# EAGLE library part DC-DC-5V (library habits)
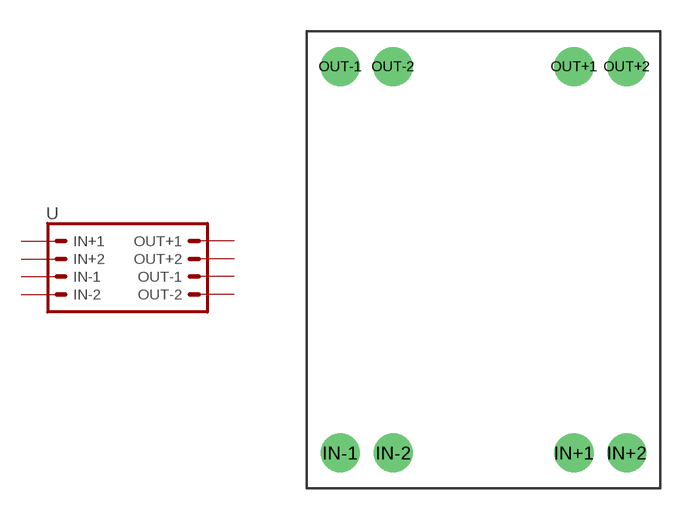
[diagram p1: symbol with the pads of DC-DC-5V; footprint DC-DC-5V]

Designator prefix U

## DC-DC-5V  [DC-DC-5V]
IN+1  IN+1  pas
IN+2  IN+2  pas
IN-1  IN-1  pas
IN-2  IN-2  pas
OUT+1  OUT+1  pas
OUT+2  OUT+2  pas
OUT-1  OUT-1  pas
OUT-2  OUT-2  pas

## Footprint DC-DC-5V (pad centres in mm)
Plated Through Hole - 2x4 Specifications: Pin count:8 Pin pitch:0.1" Example device(s): CONN_04x2
drill 1.016 pad 1.88: IN+1 4.35,-9.3; IN+2 6.89,-9.3; IN-1 -6.89,-9.3; IN-2 -4.33,-9.3; OUT+1 4.35,9.3; OUT+2 6.89,9.3; OUT-1 -6.89,9.3; OUT-2 -4.35,9.3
